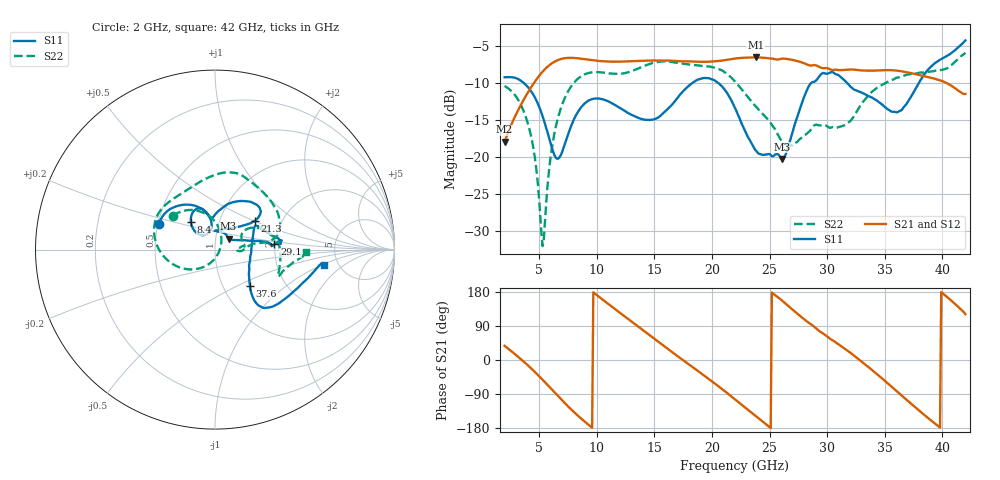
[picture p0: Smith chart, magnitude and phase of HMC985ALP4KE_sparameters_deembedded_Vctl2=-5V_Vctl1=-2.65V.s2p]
!s2p File: Measurements: S11, S21, S12, S22
# GHz S dB R 50.0
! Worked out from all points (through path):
!   401 points, 2 GHz to 42 GHz, reference 50 ohm
!   highest |S21| = -6.56 dB at 23.8 GHz (marker M1); lowest = -17.9 dB at 2 GHz (marker M2)
!   lowest |S11| = -20.2 dB at 26.1 GHz (marker M3), VSWR 1.22, Z = 57.7 + j7.13 ohm
!   |S11| at or under -10 dB: 3.662 GHz to 18.31 GHz (14.65 GHz wide, 133 % of centre); 20.54 GHz to 28.62 GHz (8.078 GHz wide, 32.9 % of centre); 31.73 GHz to 37.96 GHz (6.231 GHz wide, 17.9 % of centre)
!   |S22| runs from -32.0 to -5.9 dB; largest |S21 - S12| = 0.00056
!   S11 on the Smith chart (normalised r, x): 2 GHz: 0.50, +0.17; 8.4 GHz: 0.73, +0.23; 21.3 GHz: 1.46, +0.50; 29.1 GHz: 1.98, +0.13; 37.6 GHz: 1.33, -0.59; 42 GHz: 3.82, -1.07
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2  -9.23 155.3  -17.92 37.4  -17.93 37.4  -10.40 141.3
4.1  -10.70 120.8  -11.08 -16.3  -11.08 -16.3  -15.91 91.4
4.7  -12.18 109.6  -9.66 -33.7  -9.66 -33.7  -20.92 68.5
5.3  -14.48 100.2  -8.48 -52.2  -8.48 -52.2  -31.99 -15.2
6.5  -20.15 114.6  -7.00 -91.0  -7.01 -91.0  -15.50 -138.8
8.4  -13.82 131.3  -6.69 -147.9  -6.69 -147.9  -9.38 170.0
8.7  -13.17 127.9  -6.75 -156.0  -6.75 -156.0  -9.05 164.3
10.4  -12.16 111.3  -7.07 161.9  -7.07 161.9  -8.58 139.1
12.4  -13.73 102.4  -7.11 115.6  -7.12 115.6  -8.69 114.1
15.4  -14.59 91.9  -6.99 46.6  -6.99 46.7  -7.15 78.2
18.2  -10.12 60.3  -7.11 -15.9  -7.11 -15.9  -7.55 53.9
21.3  -11.32 35.9  -6.87 -86.7  -6.88 -86.7  -8.78 14.6
22  -13.34 39.3  -6.71 -103.8  -6.72 -103.8  -9.80 9.7
23.8  -19.09 77.0  -6.56 -147.7  -6.56 -147.7  -13.15 8.6
26.1  -20.24 39.0  -6.73 156.6  -6.73 156.6  -17.88 -2.7
28.7  -9.91 4.0  -7.63 92.1  -7.64 92.2  -15.99 7.5
29.1  -9.57 5.2  -7.66 81.8  -7.67 81.9  -15.63 6.0
32.5  -10.98 25.3  -8.23 7.4  -8.23 7.4  -14.03 33.0
35.4  -13.67 7.1  -8.27 -65.3  -8.27 -65.2  -9.77 14.5
37.6  -10.99 -46.4  -8.78 -123.5  -8.79 -123.5  -8.71 -5.0
39.6  -7.09 -46.7  -9.54 -173.6  -9.55 -173.5  -8.36 -22.9
42  -4.28 -8.3  -11.48 120.8  -11.49 120.9  -5.93 -1.2
